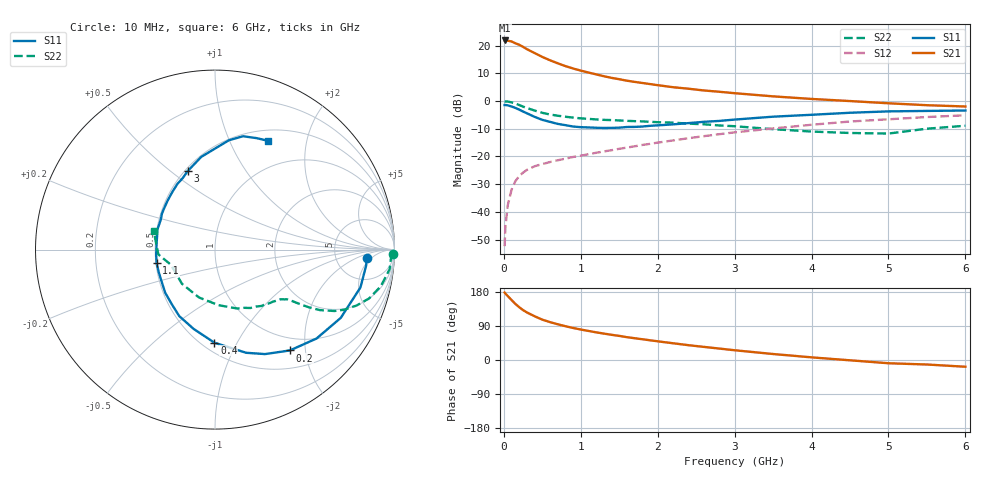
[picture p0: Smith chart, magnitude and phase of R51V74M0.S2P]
! SIEMENS Small Signal Semiconductors
! BFR183
! Si NPN RF Bipolar Junction Transistor in SOT23
! VCE = 1.75 V  IC = 4 mA
! Common Emitter S-Parameters:  May  1996
# GHz  S  MA  R  50
!  f  S11  S21  S12  S22
! GHz  MAG  ANG  MAG  ANG  MAG  ANG  MAG  ANG
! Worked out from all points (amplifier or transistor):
!   36 points, 10 MHz to 6 GHz, reference 50 ohm
!   highest |S21| = 21.9 dB at 10 MHz (marker M1)
!   |S21| within 3 dB of that: start of sweep to 291.7 MHz
!   unconditionally stable (mu >= 1): 1.119 GHz to 2.762 GHz
!   at 250 MHz: K = 0.37, MSG = 22.7 dB, |S12| = -25.8 dB
!   at 1.4 GHz: K = 1.07, MAG = 11.5 dB, |S12| = -17.7 dB
!   at 6 GHz: K = 0.90, MSG = 1.6 dB, |S12| = -5.1 dB
!   S11 on the Smith chart (normalised r, x): 10 MHz: 11, -3; 200 MHz: 0.78, -1.71; 400 MHz: 0.57, -0.81; 1.1 GHz: 0.50, -0.09; 3 GHz: 0.52, +0.57; 6 GHz: 0.63, +1.40
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0.01  0.8459 -3.0  12.4 178.0  0.0024 90.8  0.9916 -1.3
0.02  0.847 -5.9  12.24 175.4  0.0052 90.2  0.9818 -2.5
0.05  0.8373 -14.6  12.27 168.9  0.013 84.2  0.9793 -6.4
0.1  0.7972 -28.5  11.91 158.3  0.025 76.1  0.946 -12.5
0.15  0.752 -41.2  11.02 148.0  0.0358 69.1  0.9005 -17.6
0.2  0.6998 -53.4  10.37 139.3  0.0443 65.0  0.8474 -21.6
0.25  0.6455 -64.4  9.504 131.7  0.051 60.0  0.793 -25.0
0.3  0.6005 -73.2  8.642 125.5  0.0572 57.8  0.7486 -27.2
0.4  0.5184 -90.4  7.345 115.4  0.0664 54.1  0.6737 -30.0
0.5  0.4575 -105.1  6.251 106.5  0.0729 52.2  0.6127 -31.6
0.6  0.4209 -118.2  5.441 100.0  0.0792 51.6  0.5714 -32.5
0.7  0.3871 -128.7  4.804 94.3  0.0853 51.7  0.5435 -33.1
0.9  0.3467 -149.0  3.87 84.5  0.0978 52.4  0.5024 -34.1
1.1  0.334 -166.8  3.269 76.7  0.1098 53.8  0.4764 -35.6
1.3  0.3265 178.9  2.805 69.7  0.123 54.7  0.4576 -37.2
1.6  0.3401 160.9  2.327 60.2  0.1445 55.5  0.4392 -40.9
2.2  0.3792 134.3  1.776 44.2  0.1943 55.0  0.4074 -50.4
3  0.4627 109.3  1.385 25.7  0.2718 49.8  0.3511 -69.3
3.5  0.5219 98.5  1.215 15.8  0.3204 44.5  0.3104 -86.3
4.5  0.6144 82.7  0.999 -0.8  0.4269 32.4  0.265 -134.0
5.5  0.663 69.5  0.841 -11.9  0.5143 19.6  0.3169 -175.2
6  0.6744 64.0  0.797 -17.8  0.5531 11.2  0.358 162.8
